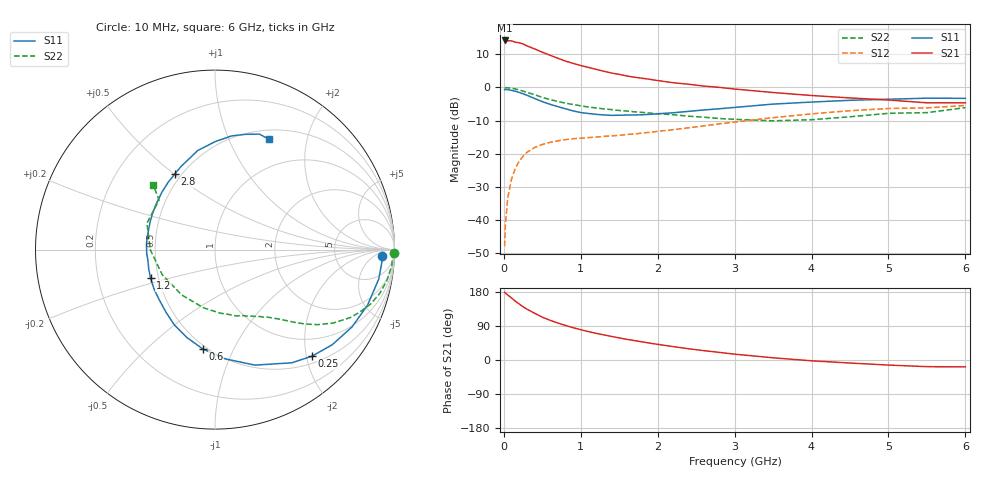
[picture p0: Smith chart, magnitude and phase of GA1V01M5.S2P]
! Infineon Technologies  Discrete & RF Semiconductors
! BF775
! Si NPN RF Bipolar Junction Transistor in SOT23
! VCE = 1 V  IC = 1.5 mA
! Common Emitter S-Parameters:  May  1996
# GHz  S  MA  R  50
!  f  S11  S21  S12  S22
! GHz  MAG  ANG  MAG  ANG  MAG  ANG  MAG  ANG
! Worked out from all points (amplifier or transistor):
!   36 points, 10 MHz to 6 GHz, reference 50 ohm
!   highest |S21| = 14.2 dB at 10 MHz (marker M1)
!   |S21| within 3 dB of that: start of sweep to 444.3 MHz
!   unconditionally stable (mu >= 1): 1.194 GHz to end of sweep
!   at 250 MHz: K = 0.26, MSG = 17.0 dB, |S12| = -20.8 dB
!   at 1.4 GHz: K = 1.12, MAG = 7.4 dB, |S12| = -14.6 dB
!   at 6 GHz: K = 1.07, MAG = -1.2 dB, |S12| = -5.4 dB
!   S11 on the Smith chart (normalised r, x): 10 MHz: 22, -11; 250 MHz: 0.63, -2.11; 600 MHz: 0.48, -0.76; 1.2 GHz: 0.45, -0.17; 2.8 GHz: 0.46, +0.50; 6 GHz: 0.62, +1.42
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0.01  0.9297 -2.1  5.134 178.8  0.004 88.4  0.9966 -1.0
0.02  0.9328 -4.1  5.066 176.6  0.0082 86.2  0.9897 -2.0
0.05  0.9269 -10.2  5.084 171.8  0.0212 84.6  0.9893 -5.1
0.1  0.9046 -20.0  5.065 163.7  0.0413 77.6  0.9733 -10.2
0.15  0.8767 -29.4  4.837 155.1  0.0603 72.1  0.9492 -15.0
0.2  0.8415 -39.0  4.735 147.8  0.077 67.0  0.9191 -19.2
0.25  0.803 -47.7  4.545 140.6  0.0912 61.7  0.8803 -23.2
0.3  0.7623 -55.8  4.253 134.2  0.1044 57.9  0.8446 -26.6
0.4  0.6812 -70.9  3.824 123.4  0.1241 50.9  0.7763 -31.8
0.5  0.6114 -84.7  3.41 113.0  0.1376 45.6  0.7095 -36.1
0.6  0.5572 -97.1  3.072 104.9  0.1481 41.6  0.6568 -39.2
0.8  0.4766 -118.4  2.507 91.2  0.1627 36.5  0.5804 -43.6
0.9  0.4433 -128.0  2.315 85.3  0.1681 35.1  0.5529 -45.4
1.1  0.4044 -147.2  2.007 75.0  0.175 33.5  0.5068 -49.1
1.2  0.3927 -156.2  1.88 70.3  0.1781 32.8  0.4896 -50.8
1.6  0.3833 174.7  1.49 54.4  0.1945 33.3  0.4398 -57.9
2.2  0.4143 142.5  1.18 35.4  0.23 35.5  0.3881 -72.2
2.8  0.4768 118.1  1.004 20.1  0.2821 35.1  0.3399 -92.8
3.5  0.5609 99.8  0.839 5.8  0.3498 30.2  0.3134 -126.5
4.5  0.6401 81.7  0.695 -8.0  0.4459 18.4  0.3608 -180.0
5.5  0.6892 69.0  0.586 -17.6  0.492 3.9  0.4167 138.4
6  0.6845 63.8  0.586 -18.1  0.534 -0.2  0.4957 133.8
